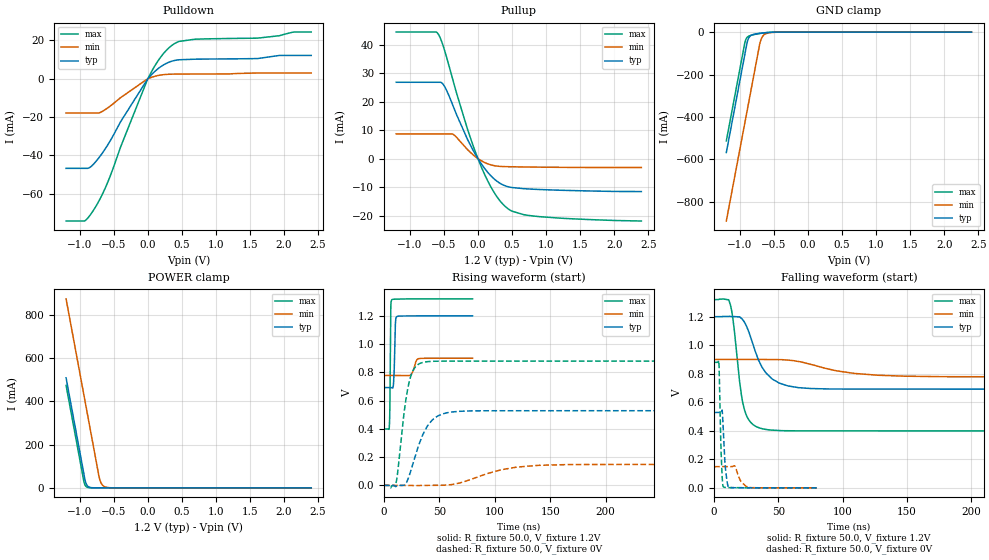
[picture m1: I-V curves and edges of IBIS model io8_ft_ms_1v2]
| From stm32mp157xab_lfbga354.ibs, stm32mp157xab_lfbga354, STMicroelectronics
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[Model]   io8_ft_ms_1v2
Model_type I/O
Polarity   Non-Inverting
Enable   Active-Low
| CAP_THRESHOLD on pad IOFT is "UDTCAPC" :
| Rising=20.00f vddiom   Falling=80.00f vddiom
| C_comp min and max val. don't necessarily correlate with the min and max pvt
| but are the smallest and greatest pad capacitance found.
| var   typ   min   max
C_comp   3.10955pF  3.08200pF  3.12755pF
|C_comp_pullup   1.83575pF  1.59875pF  1.76540pF
|C_comp_pulldown   1.27380pF  1.48325pF  1.36215pF
Vinl = 360.0mV
Vinh = 792.0mV
Vmeas = 600.0mV   | Reference voltage for timing measurements
Cref  = 50.0pF   | Timing specification test load capacitance value
Rref  = 100.0MOhm   | Timing specification test load resistance value
Vref  = 0V   | Timing specification test load voltage
[Model Spec]
| TIME_THRESHOLD on pin ZIV11 is "CMOS" :
| Rising=40.00f vdd   Falling=60.00f vdd
Vinl 463.60000mV 362.60000mV 506.60000mV
Vinh 741.40000mV 545.40000mV 817.40000mV
| variable   typ   min   max
[Temperature Range] 25.0 140.0 -40.0
| variable   typ   min   max
[Voltage Range] 1.2V 900.0mV 1.32V
| variable   typ   min   max
[POWER Clamp Reference] 1.2V 900.0mV 1.32V
| variable   typ   min   max
[GND Clamp Reference] 0V 0V 0V
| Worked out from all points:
|   slope of the pulldown table from 0 to 0.18 V, typ, clamps not added: 30 ohm
|   slope of the pullup table from 0 to 0.18 V, typ, clamps not added: 31.1 ohm
|   GND clamp passes 1 mA (typ) near -0.52 V on its own axis
|   POWER clamp passes 1 mA (typ) near -0.83 V on its own axis
|   rising waveform, R_fixture 50.0, V_fixture 1.2V: 20-80 % time 986ps typ, 2.95ns min, 507ps max; typ from 0.692 V to 1.2 V
|   falling waveform, R_fixture 50.0, V_fixture 1.2V: 20-80 % time 14.9ns typ, 38.1ns min, 7.29ns max; typ from 1.2 V to 0.692 V
|   rising waveform, R_fixture 50.0, V_fixture 0V: 20-80 % time 15.1ns typ, 38.2ns min, 8.4ns max; typ from 0 V to 0.528 V
|   falling waveform, R_fixture 50.0, V_fixture 0V: 20-80 % time 2.15ns typ, 4.87ns min, 1.52ns max; typ from 0.528 V to 0 V
[POWER Clamp]
-1.2V     508.8mA    874.1mA    473.5mA
-940mV    66.83mA    432.1mA    31.5mA
-930mV    49.83mA    415.1mA    19.15mA
-910mV    22.88mA    381.1mA    7.077mA
-880mV    7.117mA    330.1mA    1.59mA
-830mV    1.017mA    245.1mA    132uA
-720mV    14.05uA    58.12mA    554nA
-690mV    4.373uA    25.03mA    124.7nA
-650mV    922.4nA    8.136mA    17.22nA
-600mV    132.5nA    1.998mA    1.555nA
-490mV    2.763nA    90.9uA     103.5pA
2.4V      0A         0A         0A
[GND Clamp]
-1.2V     -567.2mA   -889.7mA   -512.2mA
-930mV    -108.2mA   -430.7mA   -53.23mA
-920mV    -91.21mA   -413.7mA   -40.49mA
-890mV    -43.51mA   -362.7mA   -23.59mA
-860mV    -22.57mA   -311.7mA   -17.89mA
-810mV    -12.11mA   -226.7mA   -13.23mA
-710mV    -6.053mA   -57.05mA   -7.064mA
-680mV    -4.908mA   -27.37mA   -5.632mA
-640mV    -3.605mA   -11.51mA   -3.985mA
-560mV    -1.665mA   -3.218mA   -1.61mA
-360mV    -34.72uA   -209.4uA   -9.248uA
2.4V      3.381nA    1.198uA    162.5pA
| variable   typ   min   max
[Pullup Reference] 1.2V 900.0mV 1.32V
| variable   typ   min   max
[Pulldown Reference] 0V 0V 0V
[Pullup]
-1.2V     26.81mA    8.665mA    44.46mA
-620mV    26.81mA    8.665mA    44.46mA
-580mV    26.81mA    8.665mA    43.65mA
-500mV    25.73mA    8.665mA    38.8mA
-360mV    18.22mA    8.447mA    26.96mA
-150mV    6.588mA    3.069mA    10.09mA
10mV      -383.3uA   -162.2uA   -605.9uA
220mV     -6.749mA   -2.384mA   -11.2mA
430mV     -9.803mA   -2.842mA   -17.41mA
670mV     -10.56mA   -2.945mA   -19.69mA
900mV     -10.86mA   -3.008mA   -20.39mA
2.4V      -11.58mA   -3.134mA   -21.93mA
[Pulldown]
-1.2V     -46.7mA    -17.86mA   -74.13mA
-930mV    -46.7mA    -17.86mA   -74.13mA
-860mV    -46.38mA   -17.86mA   -71.67mA
-770mV    -43.45mA   -17.86mA   -66.94mA
-580mV    -33.98mA   -14.99mA   -53.18mA
0V        0A         0A         0A
180mV     6.001mA    1.854mA    10.79mA
350mV     9.086mA    2.357mA    17.24mA
460mV     9.857mA    2.4mA      19.42mA
690mV     10.15mA    2.431mA    20.56mA
1.61V     10.48mA    2.965mA    21.11mA
2.4V      12.11mA    2.965mA    24.31mA
[Ramp]
dV/dt_r 316.98748mV/15.10494ns 89.07933mV/38.19342ns 527.83986mV/8.40308ns
dV/dt_f 304.65085mV/14.85133ns 73.18319mV/38.10995ns 552.41129mV/7.28486ns
R_load = 50.0
| Removed startup time: 0s 0s 0s  .
| Removed end time: 79.9ns.
[Rising Waveform]
R_fixture   = 50.0
V_fixture   = 1.2V
V_fixture_min = 900.0mV
V_fixture_max = 1.32V
0s        692.2mV    778mV      399.3mV
4.9ns     692.2mV    778mV      421.8mV
5.4ns     692.2mV    778mV      595.4mV
6ns       692.3mV    778mV      1.21V
7ns       691.6mV    778mV      1.313V
8.7ns     730.8mV    778mV      1.317V
10.3ns    1.139V     778mV      1.318V
11.5ns    1.194V     778mV      1.319V
31.2ns    1.2V       896.8mV    1.32V
79.9ns    1.2V       899.8mV    1.32V
| Removed startup time: 0s 0s 0s  .
| Removed end time: 799.9ns.
[Falling Waveform]
R_fixture   = 50.0
V_fixture   = 1.2V
V_fixture_min = 900.0mV
V_fixture_max = 1.32V
0s        1.2V       900mV      1.32V
12.8ns    1.202V     900mV      1.279V
15.3ns    1.201V     899.9mV    1.14V
21ns      1.19V      900.7mV    663.8mV
25.2ns    1.134V     900.5mV    507.1mV
34.2ns    902.3mV    900.4mV    423.4mV
43.5ns    777.8mV    900mV      405.4mV
65.8ns    702.5mV    885.6mV    399.5mV
147.7ns   692.2mV    783mV      399.3mV
799.9ns   692.2mV    778mV      399.3mV
| Removed startup time: 0s 0s 0s  .
| Removed end time: 799.9ns.
[Rising Waveform]
R_fixture   = 50.0
V_fixture   = 0V
V_fixture_min = 0V
V_fixture_max = 0V
0s        51.25nV    1.017uV    136.8nV
10.6ns    -9.66mV    1.096uV    8.611mV
18.4ns    2.703mV    -103.3nV   528.7mV
22.9ns    70.74mV    -86.19uV   736.8mV
28.6ns    218mV      -1.994mV   841mV
38ns      402.5mV    -95.15uV   874.4mV
60.9ns    519.3mV    5.498mV    879.6mV
106.1ns   528.1mV    111mV      879.7mV
166.1ns   528.2mV    147.1mV    879.7mV
799.9ns   528.3mV    148.5mV    879.7mV
| Removed startup time: 0s 0s 0s  .
| Removed end time: 79.9ns.
[Falling Waveform]
R_fixture   = 50.0
V_fixture   = 0V
V_fixture_min = 0V
V_fixture_max = 0V
0s        528.3mV    148.5mV    879.7mV
3.7ns     528.3mV    148.5mV    889.5mV
5.5ns     529.1mV    148.5mV    244.5mV
6.4ns     535.2mV    148.5mV    57.28mV
7.2ns     395.5mV    148.5mV    7.526mV
8.8ns     139.5mV    148.5mV    2.482mV
11.5ns    3.625mV    148.5mV    1.517mV
16.2ns    788.8uV    153mV      757.8uV
27.1ns    487.2uV    2.986mV    124.8uV
79.9ns    1.487uV    123.5uV    2.188uV
